(*此PLC项目为FB_XmlSrvReadByName对应例程,FB_XmlSrvWriteByName请打开名称为XmlWriteByName的PLC项目*)
PROGRAM MAIN
VAR
	ST_XmlWrite2: ST_XmlTest2;
	FB_XmlReadByName: FB_XmlSrvReadByName;
	b_Execute: BOOL;
	sSymName: T_MaxString :='MAIN.ST_XmlWrite2';		
	sFilePath: T_MaxString:='C:\temp\Test.xml';		
	sXPath: T_MaxString:='/dataentry/MAIN.ST_XmlWrite2';
END_VAR

FB_XmlReadByName(
	sNetId:= , 
	ePath:= PATH_GENERIC, 
	nMode:= XMLSRV_ADDMISSING, 
	sSymName:= sSymName, 
	sFilePath:= sFilePath, 
	sXPath:= sXPath, 
	bExecute:= b_Execute, 
	tTimeout:= , 
	bBusy=> , 
	bError=> , 
	nErrId=> );

END_PROGRAM
